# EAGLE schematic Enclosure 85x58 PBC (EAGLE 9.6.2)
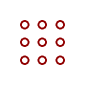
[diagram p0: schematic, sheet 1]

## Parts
U$1  PROTO-28X18-C  [PROTO-28X18-C]

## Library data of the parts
U$1 = digitalconcepts:PROTO-28X18-C: 28 x 18 Prototyping board to fit an 85 x 58 enclosure, with external connector cut-outs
